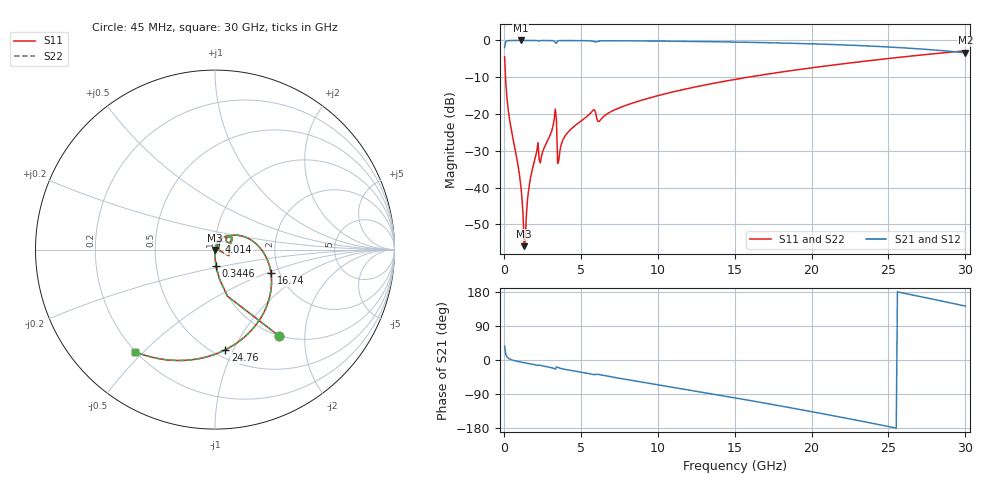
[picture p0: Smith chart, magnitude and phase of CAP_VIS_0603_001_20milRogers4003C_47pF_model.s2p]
! S-parameter model data by Modelithics Inc.  support@modelithics.com  813-866-6335  Tampa FL USA
! S-Parameter data specifications:
! Substrate: 20-mil Rogers 4003C, substrate thickness, H=0.508mm, Dielectric constant, Er=3.75
! PCB Mounting Pad Footprint: Pad width, PadW=0.90mm , Pad length, PadL=1.00mm , Pad gap, PadG (edge-to-edge)=1.00mm , Reference planes=3.0mm apart
! Created Wed Nov 18 13:29:01 2015
# hz S ma R 50
! 2 Port Network Data from SP1.SP block
! freq  magS11  angS11  magS21  angS21  magS12  angS12  magS22  angS22
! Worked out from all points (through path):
!   401 points, 45 MHz to 30 GHz, reference 50 ohm
!   highest |S21| = -0.01 dB at 1.093 GHz (marker M1); lowest = -3.3 dB at 30 GHz (marker M2)
!   group delay of S21, straight-line fit = 20.2 ps
!   lowest |S11| = -55.9 dB at 1.318 GHz (marker M3), VSWR 1.00, Z = 50.1 - j0.132 ohm
!   |S11| at or under -10 dB: 104.6 MHz to 15.86 GHz (15.75 GHz wide, 197 % of centre)
!   |S22| runs from -55.9 to -2.8 dB; largest |S21 - S12| = 0
!   S11 on the Smith chart (normalised r, x): 45 MHz: 0.99, -1.49; 344.6 MHz: 1.00, -0.18; 4.014 GHz: 1.05, +0.10; 16.74 GHz: 1.80, -0.54; 24.76 GHz: 0.57, -0.93; 30 GHz: 0.20, -0.47
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4.5e7  0.5989 -53.4  0.8006 36.5  0.8006 36.5  0.5989 -53.4
3.4455e8  0.09115 -86.3  0.9952 3.3  0.9952 3.3  0.09115 -86.3
1.093425e9  0.01082 -90.2  0.9989 -5.4  0.9989 -5.4  0.01082 -90.2
1.2432e9  0.004317 -82.6  0.9988 -6.6  0.9988 -6.6  0.004317 -82.6
1.318088e9  0.001605 -54.8  0.9988 -7.2  0.9988 -7.2  0.001605 -54.8
1.467862e9  0.004563 67.0  0.9987 -8.3  0.9987 -8.3  0.004563 67.0
1.692525e9  0.01229 74.0  0.9985 -10.0  0.9985 -10.0  0.01229 74.0
2.066962e9  0.02657 72.5  0.9973 -12.9  0.9973 -12.9  0.02657 72.5
2.4414e9  0.02685 69.1  0.9966 -15.0  0.9966 -15.0  0.02685 69.1
3.265162e9  0.08374 57.1  0.9814 -22.7  0.9814 -22.7  0.08374 57.1
3.6396e9  0.03165 57.9  0.9936 -21.8  0.9936 -21.8  0.03165 57.9
4.014038e9  0.05175 62.1  0.9957 -25.0  0.9957 -25.0  0.05175 62.1
5.062462e9  0.08181 55.5  0.9933 -32.5  0.9933 -32.5  0.08181 55.5
5.73645e9  0.1093 45.1  0.9799 -37.7  0.9799 -37.7  0.1093 45.1
6.260662e9  0.08271 42.2  0.9835 -39.0  0.9835 -39.0  0.08271 42.2
1.007992e10  0.1793 23.4  0.9799 -65.6  0.9799 -65.6  0.1793 23.4
1.50225e10  0.2955 -10.6  0.9503 -99.9  0.9503 -99.9  0.2955 -10.6
1.674491e10  0.3386 -22.9  0.9354 -112.3  0.9354 -112.3  0.3386 -22.9
2.003996e10  0.4254 -47.2  0.8985 -136.6  0.8985 -136.6  0.4254 -47.2
2.475788e10  0.5609 -84.1  0.8197 -173.5  0.8197 -173.5  0.5609 -84.1
2.505742e10  0.57 -86.5  0.8133 -176.0  0.8133 -176.0  0.57 -86.5
3e10  0.7227 -128.2  0.6803 142.3  0.6803 142.3  0.7227 -128.2
